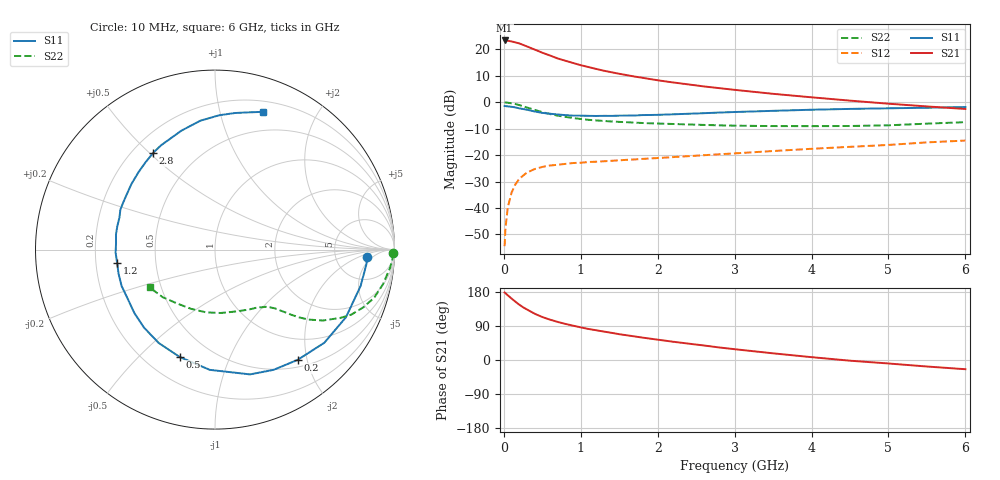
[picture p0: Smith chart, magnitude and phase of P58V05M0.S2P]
! SIEMENS Small Signal Semiconductors
! BFP183
! Si NPN RF Bipolar Junction Transistor in SOT143
! VCE = 8 V  IC = 5 mA
! Common Emitter S-Parameters:  March  1996
# GHz  S  MA  R  50
!  f  S11  S21  S12  S22
! GHz  MAG  ANG  MAG  ANG  MAG  ANG  MAG  ANG
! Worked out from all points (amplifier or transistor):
!   36 points, 10 MHz to 6 GHz, reference 50 ohm
!   highest |S21| = 23.4 dB at 10 MHz (marker M1)
!   |S21| within 3 dB of that: start of sweep to 363.5 MHz
!   unconditionally stable (mu >= 1): 1.646 GHz to 5.775 GHz
!   at 250 MHz: K = 0.20, MSG = 24.7 dB, |S12| = -27.7 dB
!   at 1.4 GHz: K = 0.91, MSG = 16.7 dB, |S12| = -22.1 dB
!   at 6 GHz: K = 0.96, MSG = 6.0 dB, |S12| = -14.5 dB
!   lowest NFmin = 1.15 dB at 450 MHz
!   S11 on the Smith chart (normalised r, x): 10 MHz: 11, -3; 200 MHz: 0.61, -1.84; 500 MHz: 0.34, -0.67; 1.2 GHz: 0.29, -0.06; 2.8 GHz: 0.28, +0.51; 6 GHz: 0.30, +1.36
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0.01  0.8493 -2.6  14.75 178.1  0.0019 86.0  0.992 -1.2
0.02  0.8472 -5.6  14.63 176.6  0.0039 85.2  0.9916 -2.4
0.05  0.8363 -14.0  14.58 170.9  0.0101 85.6  0.9814 -5.8
0.1  0.8212 -27.3  14.13 162.2  0.0195 75.2  0.956 -11.6
0.15  0.8003 -40.4  13.55 153.9  0.028 68.7  0.9266 -16.8
0.2  0.7679 -53.1  12.99 146.1  0.0355 63.3  0.8864 -21.3
0.25  0.7452 -64.0  12.16 139.1  0.041 58.1  0.8415 -25.5
0.3  0.7222 -74.3  11.39 133.4  0.0467 53.8  0.7967 -28.5
0.4  0.6706 -92.5  9.938 122.2  0.0546 47.0  0.7195 -33.3
0.5  0.6297 -108.2  8.649 113.4  0.0599 41.8  0.6509 -36.8
0.6  0.6074 -121.1  7.662 106.5  0.0637 38.3  0.5987 -39.0
0.7  0.5877 -132.3  6.737 100.5  0.0658 35.7  0.5588 -40.5
0.9  0.5581 -150.8  5.531 90.6  0.071 32.4  0.5039 -42.7
1.1  0.5538 -166.1  4.635 81.9  0.0742 30.8  0.4655 -44.6
1.2  0.5504 -172.0  4.27 78.5  0.0751 30.1  0.4537 -45.6
1.7  0.5617 161.4  3.063 62.2  0.0829 30.1  0.4127 -51.2
2.2  0.5918 141.9  2.369 48.2  0.0919 30.3  0.3885 -58.3
2.8  0.6389 122.8  1.85 33.1  0.1039 30.6  0.3663 -69.4
3.5  0.6886 105.8  1.445 17.6  0.1197 29.5  0.3546 -84.8
4.5  0.7489 88.2  1.074 -1.8  0.1437 25.8  0.356 -112.0
5.5  0.7874 76.2  0.834 -17.2  0.1744 21.5  0.3941 -137.7
6  0.8121 70.9  0.747 -24.3  0.1887 17.6  0.4209 -150.0
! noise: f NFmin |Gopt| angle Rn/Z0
0.45  1.15  0.25  40  0.26
0.9  1.2  0.25  93  0.22
1.8  1.95  0.32  170  0.13
